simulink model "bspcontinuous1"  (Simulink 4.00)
settings: Solver=ode45  StartTime=0.0  StopTime=25  FixedStep=0.01  RelTol=1e-3
libraries: simulink3 x1

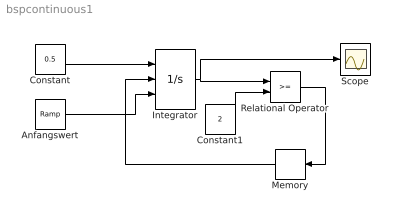
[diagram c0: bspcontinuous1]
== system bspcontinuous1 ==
  Anfangswert : simulink3/Sources/Ramp  slope=0.1  start=0  X0=0
  Constant : Constant  Value=0.5
  Constant1 : Constant  Value=2
  Integrator : Integrator  ExternalReset=rising  InitialConditionSource=external  InitialCondition=0  LimitOutput=on  UpperSaturationLimit=2  LowerSaturationLimit=-inf  ShowSaturationPort=off  ShowStatePort=off  AbsoluteTolerance=auto
  Memory : Memory  Orientation=left  X0=0  InheritSampleTime=off
  Relational Operator : RelationalOperator  Operator=>=
  Scope : Scope
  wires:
  Constant/1 -> Integrator/1
  Constant1/1 -> Relational Operator/2
  Integrator/1 -> Relational Operator/1, Scope/1
  Anfangswert/1 -> Integrator/3
  Relational Operator/1 -> Memory/1
  Memory/1 -> Integrator/2
